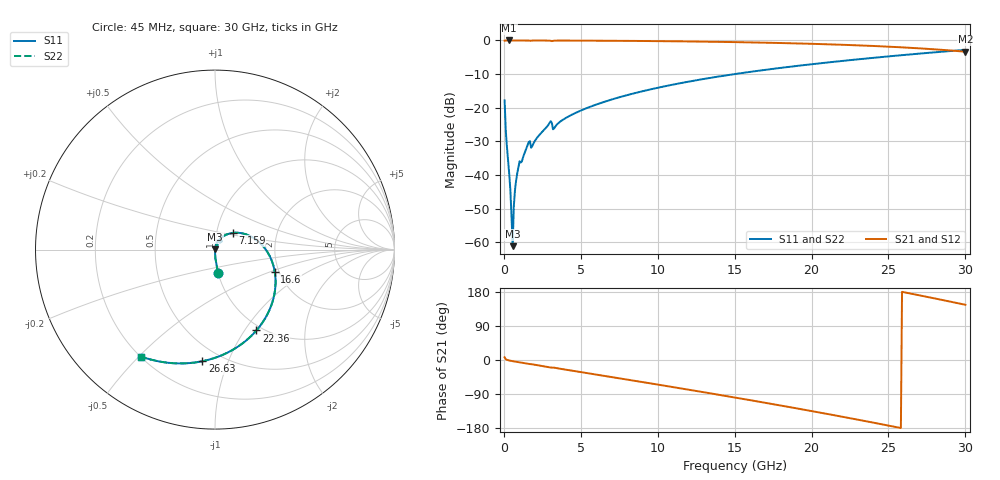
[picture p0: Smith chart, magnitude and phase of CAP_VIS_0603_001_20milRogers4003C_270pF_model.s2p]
! S-parameter model data by Modelithics Inc.  support@modelithics.com  813-866-6335  Tampa FL USA
! S-Parameter data specifications:
! Substrate: 20-mil Rogers 4003C, substrate thickness, H=0.508mm, Dielectric constant, Er=3.75
! PCB Mounting Pad Footprint: Pad width, PadW=0.90mm , Pad length, PadL=1.00mm , Pad gap, PadG (edge-to-edge)=1.00mm , Reference planes=3.0mm apart
! Created Wed Nov 18 13:33:32 2015
# hz S ma R 50
! 2 Port Network Data from SP1.SP block
! freq  magS11  angS11  magS21  angS21  magS12  angS12  magS22  angS22
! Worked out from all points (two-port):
!   401 points, 45 MHz to 30 GHz, reference 50 ohm
!   highest |S21| = 0.00 dB at 344.6 MHz (marker M1); lowest = -3.3 dB at 30 GHz (marker M2)
!   |S21| within 3 dB of the highest: start of sweep to 29.09 GHz
!   lowest |S11| = -61.2 dB at 569.2 MHz (marker M3), VSWR 1.00, Z = 50.1 + j0.0665 ohm
!   |S11| at or under -10 dB: start of sweep to 15 GHz
!   |S22| runs from -61.2 to -2.8 dB; largest |S21 - S12| = 0
!   S11 on the Smith chart (normalised r, x): 45 MHz: 1.00, -0.26; 7.159 GHz: 1.20, +0.23; 16.6 GHz: 1.90, -0.54; 22.36 GHz: 0.94, -1.13; 26.63 GHz: 0.40, -0.81; 30 GHz: 0.20, -0.51
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4.5e7  0.1287 -82.8  0.9915 7.2  0.9915 7.2  0.1287 -82.8
1.94775e8  0.02644 -88.8  0.9993 0.5  0.9993 0.5  0.02644 -88.8
3.4455e8  0.01045 -88.9  0.9995 -1.2  0.9995 -1.2  0.01045 -88.9
4.194375e8  0.00596 -87.5  0.9995 -1.9  0.9995 -1.9  0.00596 -87.5
5.692125e8  0.0008747 49.4  0.9994 -3.1  0.9994 -3.1  0.0008747 49.4
6.441e8  0.003448 76.8  0.9994 -3.6  0.9994 -3.6  0.003448 76.8
7.93875e8  0.008295 80.6  0.9992 -4.7  0.9992 -4.7  0.008295 80.6
9.4365e8  0.01314 79.6  0.9988 -5.8  0.9988 -5.8  0.01314 79.6
1.54275e9  0.02768 75.9  0.9974 -9.8  0.9974 -9.8  0.02768 75.9
1.917188e9  0.02935 73.6  0.9971 -11.9  0.9971 -11.9  0.02935 73.6
2.965612e9  0.05906 66.3  0.9934 -19.2  0.9934 -19.2  0.05906 66.3
3.34005e9  0.05245 64.9  0.9944 -20.9  0.9944 -20.9  0.05245 64.9
5.062462e9  0.09207 56.7  0.9937 -32.3  0.9937 -32.3  0.09207 56.7
7.159312e9  0.1357 43.2  0.9883 -46.0  0.9883 -46.0  0.1357 43.2
1.007992e10  0.1997 24.0  0.9768 -65.4  0.9768 -65.4  0.1997 24.0
1.50225e10  0.3167 -9.5  0.9445 -99.1  0.9445 -99.1  0.3167 -9.5
1.659514e10  0.3557 -20.5  0.9302 -110.1  0.9302 -110.1  0.3557 -20.5
2.003996e10  0.444 -45.4  0.8908 -135.0  0.8908 -135.0  0.444 -45.4
2.236148e10  0.5061 -62.9  0.8566 -152.5  0.8566 -152.5  0.5061 -62.9
2.505742e10  0.5811 -83.9  0.807 -173.5  0.807 -173.5  0.5811 -83.9
2.663006e10  0.6262 -96.5  0.7722 173.8  0.7722 173.8  0.6262 -96.5
3e10  0.7242 -124.6  0.6805 145.7  0.6805 145.7  0.7242 -124.6
